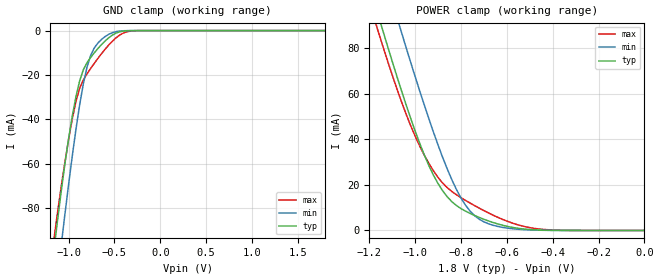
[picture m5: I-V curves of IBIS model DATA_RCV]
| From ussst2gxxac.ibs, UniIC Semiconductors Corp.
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|   Model DATA_RCV
[Model]  DATA_RCV
Model_type Input
Polarity   Non-Inverting
Vinl =   0.70000000V
Vinh =   1.10000000V
C_comp   2.5240pF   2.5060pF   2.5510pF
[Temperature Range]   25.0000   95.0000   0.0
[Voltage Range]   1.8000V   1.7000V   1.9000V
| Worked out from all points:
|   GND clamp passes 1 mA (typ) near -0.47 V on its own axis
|   POWER clamp passes 1 mA (typ) near -0.55 V on its own axis
[GND_clamp]
|Voltage   I(typ)   I(min)   I(max)
-1.8V     -341.4mA   -368.9mA   -332.4mA
-1.16V    -98.84mA   -124.9mA   -94.02mA
-1.12V    -85.23mA   -110.5mA   -81.66mA
-1.08V    -72.2mA    -96.41mA   -70.06mA
-1.04V    -59.93mA   -82.62mA   -59.18mA
-920mV    -29.77mA   -44.48mA   -31.9mA
-880mV    -22.69mA   -33.57mA   -26.06mA
-800mV    -14.49mA   -16.62mA   -19.53mA
-720mV    -10.02mA   -7.817mA   -14.76mA
-560mV    -3.159mA   -1.628mA   -6.393mA
-280mV    -8.14uA    -3.578uA   -70uA
1.8V      7.234nA    32.16nA    61.22nA
[POWER_clamp]
|Voltage   I(typ)   I(min)   I(max)
-1.8V     325.1mA    352.4mA    316.2mA
-1.16V    94.14mA    121mA      86.98mA
-1.14V    87.41mA    114.1mA    80.57mA
-1.06V    61.46mA    87.09mA    56.62mA
-980mV    38.21mA    61.22mA    37.03mA
-900mV    20.56mA    37.47mA    23.27mA
-820mV    10.96mA    18mA       15.69mA
-780mV    8.467mA    11.05mA    13.18mA
-740mV    6.55mA     6.435mA    10.88mA
-640mV    2.87mA     1.791mA    5.795mA
-480mV    290.4uA    171.3uA    911.2uA
0V        7.234nA    10.13nA    70.66nA
